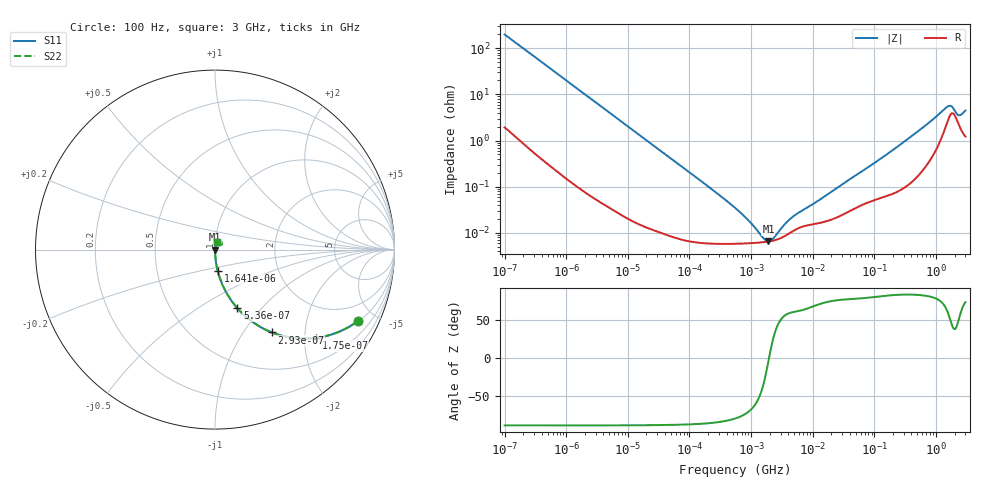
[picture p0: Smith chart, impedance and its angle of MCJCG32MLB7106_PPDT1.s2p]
! MCJCG32MLB7106_PPDT1  S-PARAMETER MODEL  ( Standard Model )
! Model Generated by TAIYO YUDEN Corporation (http://www.ty-top.com)
! Version 1.0
! TAIYO YUDEN Control No. 220601
! Copyright(c) 2015 TAIYO YUDEN CO.,LTD. All Rights Reserved.
! Product Description (link to TY-COMPAS)
! https://ds.yuden.co.jp/TYCOMPAS/or/detail?pn=MCJCG32MLB7106KPPDT1&u=M
! Products Name : Multilayer Ceramic Capacitors
! Characteristics :
!  Capacitance : 10 [uF] , Rated Voltage : 35 [V] , TCC : X7R
!  Case Size : 3.2 x 2.5 / 0.126 x 0.098 [mm/inch] , Thickness : 2.5 / 0.098 [mm/inch]
!  (Conditions: Temperature = 25 [degC] , DC Bias Voltage = 0 [V])
! External Node Assignments :
!  1  o---| |---o  2
! GND o---------o GND
! Frequency Range : 100Hz  -  3GHz  [ 401 STEP ]
# MHZ S RI R 50
! Freq[MHz].  S11 Real  S11 Imag  S21 Real  S21 Imag  S12 Real  S12 Imag  S22 Real  S22 Imag
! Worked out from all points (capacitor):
!   401 points, 100 Hz to 3 GHz, reference 50 ohm
!   read as one part in series: C = 8.01 uF near 109 Hz
!   lowest |Z| = 6.51 mohm at 1.908 MHz (marker M1)
!   series resonance near 1.954 MHz, so ESL is about 830 pH
!   S11 on the Smith chart (normalised r, x): 100 Hz: 1.04, -3.97; 175 Hz: 1.02, -2.28; 293 Hz: 1.01, -1.36; 536 Hz: 1.01, -0.75; 1.641 kHz: 1.00, -0.25; 3 GHz: 1.02, +0.09
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0.0001  0.7952 -0.3987  0.2048 0.3987  0.2048 0.3987  0.7952 -0.3987
0.000175  0.564 -0.4915  0.436 0.4915  0.436 0.4915  0.564 -0.4915
0.000293  0.3182 -0.4618  0.6818 0.4618  0.6818 0.4618  0.3182 -0.4618
0.000536  0.1245 -0.3264  0.8755 0.3264  0.8755 0.3264  0.1245 -0.3264
0.00086  0.0531 -0.2206  0.9469 0.2206  0.9469 0.2206  0.0531 -0.2206
0.001641  0.0157 -0.1206  0.9843 0.1206  0.9843 0.1206  0.0157 -0.1206
0.001788  0.0133 -0.111  0.9867 0.111  0.9867 0.111  0.0133 -0.111
0.005476  0.00169 -0.0369  0.9983 0.0369  0.9983 0.0369  0.00169 -0.0369
0.031977  0.000144 -0.00638  0.9999 0.00638  0.9999 0.00638  0.000144 -0.00638
0.547723  5.81e-05 -0.000345  0.9999 0.000345  0.9999 0.000345  5.81e-05 -0.000345
1.352413  6.17e-05 -7.86e-05  0.9999 7.86e-05  0.9999 7.86e-05  6.17e-05 -7.86e-05
1.908323  6.49e-05 -4.87e-06  0.9999 4.87e-06  0.9999 4.87e-06  6.49e-05 -4.87e-06
2.69274  7.24e-05 6.85e-05  0.9999 -6.85e-05  0.9999 -6.85e-05  7.24e-05 6.85e-05
4.711951  0.000108 0.000194  0.9999 -0.000194  0.9999 -0.000194  0.000108 0.000194
9.794414  0.000153 0.000381  0.9998 -0.000381  0.9998 -0.000381  0.000153 0.000381
175.1444  0.000685 0.00546  0.9993 -0.00546  0.9993 -0.00546  0.000685 0.00546
610.2215  0.00261 0.0189  0.9974 -0.0189  0.9974 -0.0189  0.00261 0.0189
1506.733  0.0255 0.0453  0.9745 -0.0453  0.9745 -0.0453  0.0255 0.0453
1789.813  0.0386 0.0363  0.9614 -0.0363  0.9614 -0.0363  0.0386 0.0363
2317.205  0.0231 0.0259  0.9769 -0.0259  0.9769 -0.0259  0.0231 0.0259
2525.516  0.0183 0.0303  0.9817 -0.0303  0.9817 -0.0303  0.0183 0.0303
3000  0.0139 0.0418  0.9861 -0.0418  0.9861 -0.0418  0.0139 0.0418
